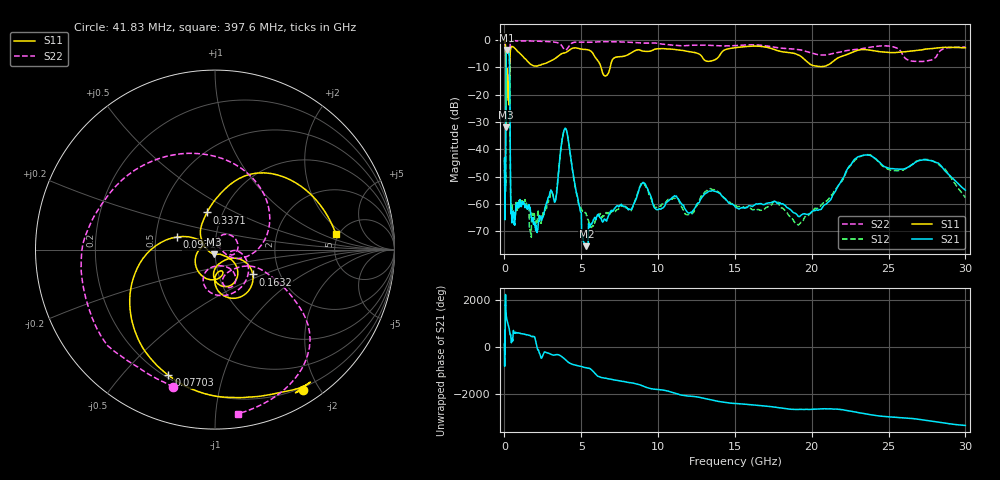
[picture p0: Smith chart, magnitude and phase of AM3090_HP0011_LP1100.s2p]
! Date/Time: Thu, Feb 28, 2019 1:56 PM
! Network Analyzer: Agilent Technologies E8364B Rev: A.07.50.67
! Sweep from 0.010 to 30.000 GHz, 1601 Points, Sweep Type: LOG
! Power Supply: 5.023 V, 0.002 A
# Hz S DB R 50
!freq MagS11 AngS11 MagS21 AngS21 MagS12 AngS12 MagS22 AngS22
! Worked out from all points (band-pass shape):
!   1601 points, 10 MHz to 30 GHz, reference 50 ohm
!   highest |S21| = -3.65 dB at 155.2 MHz (marker M1); lowest = -75.5 dB at 5.338 GHz (marker M2)
!   |S21| within 3 dB of the highest: 103.4 MHz to 320.1 MHz (216.7 MHz wide, 102 % of centre)
!   lowest |S11| = -31.9 dB at 100.9 MHz (marker M3), VSWR 1.05, Z = 49.5 - j2.47 ohm
!   |S11| at or under -10 dB: 91.57 MHz to 349.4 MHz (257.9 MHz wide, 117 % of centre); 6.288 GHz to 6.877 GHz (588.8 MHz wide, 8.94 % of centre)
!   |S22| runs from -31.6 to -0.1 dB; largest |S21 - S12| = 0.011
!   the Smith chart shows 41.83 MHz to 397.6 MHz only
!   S11 on the Smith chart (normalised r, x): 41.83 MHz: 0.17, -1.79; 77.03 MHz: 0.21, -0.67; 93.16 MHz: 0.65, +0.10; 163.2 MHz: 1.46, -0.43; 337.1 MHz: 0.84, +0.37; 397.6 MHz: 4.69, +1.55
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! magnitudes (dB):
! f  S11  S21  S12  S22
! 10 MHz  -0.3  -44.5  -45.8  -0.6
! 38.04 MHz  -0.5  -60.2  -62.3  -1.6
! 41.83 MHz  -0.7  -64.7  -63.6  -1.9
! 49.1 MHz  -0.8  -49.4  -48.5  -1.9
! 77.03 MHz  -2.5  -45.3  -46.6  -4.6
! 93.16 MHz  -13.1  -14.2  -14.2  -13.1
! 100.9 MHz  -31.9  -7.4  -7.4  -31.0
! 116.1 MHz  -13.5  -4.9  -4.9  -18.9
! 144.7 MHz  -20.7  -3.7  -3.7  -21.2
! 155.2 MHz  -14.4  -3.6  -3.6  -17.3
! 163.2 MHz  -12.0  -3.7  -3.6  -14.6
! 337.1 MHz  -13.5  -10.0  -10.0  -8.4
! 397.6 MHz  -3.4  -54.7  -53.5  -0.7
! 550.5 MHz  -2.5  -62.8  -62.4  -0.2
! 2.084 GHz  -9.5  -70.0  -66.4  -0.4
! 3.302 GHz  -6.7  -59.1  -58.4  -0.8
! 3.953 GHz  -4.6  -32.3  -32.3  -3.6
! 5.338 GHz  -3.4  -75.5  -64.3  -0.8
! 7.926 GHz  -5.6  -61.3  -61.4  -0.7
! 19.22 GHz  -5.7  -64.7  -67.3  -3.5
! 23.48 GHz  -3.5  -42.1  -42.0  -2.9
! 30 GHz  -2.8  -55.0  -57.7  -2.5
